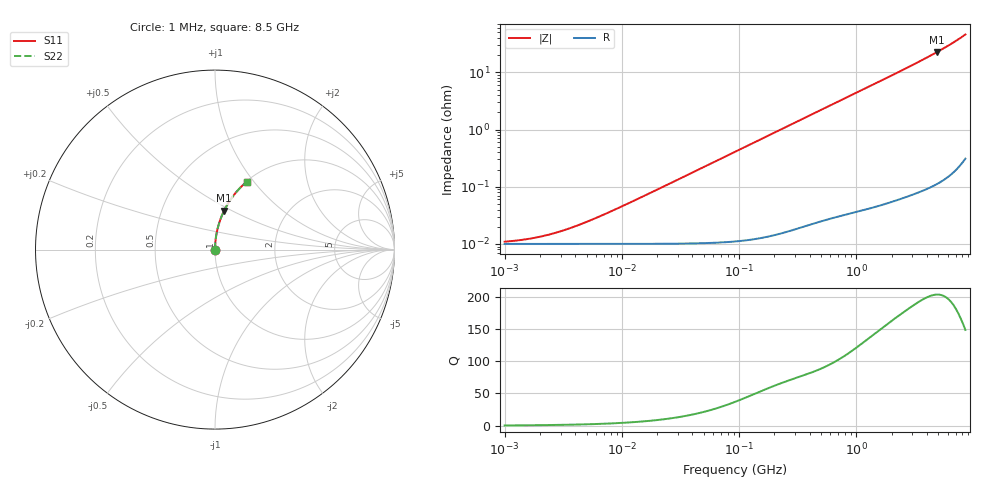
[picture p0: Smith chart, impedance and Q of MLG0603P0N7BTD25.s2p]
! S-Parameter Data Generated by TDK Corporation
! Copyright(C) 2025 TDK Corporation.
! All Rights Reserved.
! TDK P/N: MLG0603P0N7BTD25 (SMD / SMT Inductor (Coil))
! Property: L=0.7nH at 500MHz
! Size(LxWxT): 0.6x0.3x0.3mm
! Model Type: s2p (Touchstone File Format Version 1.0)
! Frequency: DC=Yes Start=1MHz Stop=8500MHz 198points Log-sweep
! Model Generated on Feb. 6, 2025
! Terms and conditions regarding TDK Simulation Models:
! 1)This simulation model is being provided solely for informational
!  purposes. Please refer to the specifications of the products in
!  terms of detailed characteristics of such products.
! 2)In no event shall TDK Corporation of any of its subsidiaries be
!  liable for any loss or damage arising, directly or indirectly,
!  from any information contained in this simulation model, including,
!  but not limited to loss or damages arising from any inaccuracies,
!  omissions or errors in connection with such information.
! 3)Any and all copyrights on this simulation model are owned by
!  TDK Corporation.  Duplication or redistribution of this simulation
!  model without prior written permission from TDK Corporation
!  is prohibited.
! 4)This simulation model is subject to any modification or change
!  without any prior notice.
! 5)Neither TDK Corporation nor any of its subsidiaries shall make any
!  warranty, express or implied, including but not limited to the
!  correctness, implied warranties of merchantability and fitness for
!  a particular purpose with respect to this simulation models.
! 6)The use of this simulation model shall be deemed to have consented
!  to the terms and conditions hereof.
! Port Assignments:
!  1 ---@@@--- 2
! Applicable Conditions:
!  Temperature = 25 degC
!  DC Bias Current = 0 A
!  Small Signal Operation
# Hz S MA R 50
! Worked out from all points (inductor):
!   197 points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, 1 MHz to 8.5 GHz, reference 50 ohm
!   read as one part in series: L = 704 pH near 6.951 MHz
!   highest Q = 203 at 4.885 GHz (marker M1), where L = 742 pH
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1000000  0.0001093 23.9  0.9999 -0.0  0.9999 -0.0  0.0001093 23.9
1515069  0.0001204 33.8  0.9999 -0.0  0.9999 -0.0  0.0001204 33.8
1822320  0.0001285 38.9  0.9999 -0.0  0.9999 -0.0  0.0001285 38.9
2191881  0.0001393 44.1  0.9999 -0.0  0.9999 -0.0  0.0001393 44.1
2636387  0.0001536 49.4  0.9999 -0.0  0.9999 -0.0  0.0001536 49.4
3171038  0.0001723 54.5  0.9999 -0.0  0.9999 -0.0  0.0001723 54.5
4587603  0.0002263 63.8  0.9999 -0.0  0.9999 -0.0  0.0002263 63.8
6051655  0.0002858 69.5  0.9999 -0.0  0.9999 -0.0  0.0002858 69.5
8360083  0.0003832 74.8  0.9999 -0.0  0.9999 -0.0  0.0003832 74.8
2.10461e7  0.0009366 83.8  0.9999 -0.1  0.9999 -0.1  0.0009366 83.8
9.219544e7  0.004079 88.2  0.9999 -0.2  0.9999 -0.2  0.004079 88.2
4.229561e8  0.01861 88.2  0.9996 -1.1  0.9996 -1.1  0.01861 88.2
1.016736e9  0.04459 87.0  0.9986 -2.6  0.9986 -2.6  0.04459 87.0
1.940355e9  0.0853 84.8  0.9958 -4.9  0.9958 -4.9  0.0853 84.8
2.559585e9  0.113 83.2  0.993 -6.5  0.993 -6.5  0.113 83.2
3.224109e9  0.1432 81.5  0.9889 -8.2  0.9889 -8.2  0.1432 81.5
4.061159e9  0.1821 79.2  0.9824 -10.5  0.9824 -10.5  0.1821 79.2
4.884749e9  0.2218 76.9  0.974 -12.8  0.974 -12.8  0.2218 76.9
5.87536e9  0.2715 74.0  0.9611 -15.8  0.9611 -15.8  0.2715 74.0
6.748056e9  0.3176 71.2  0.9465 -18.5  0.9465 -18.5  0.3176 71.2
7.750377e9  0.3735 67.7  0.9254 -21.9  0.9254 -21.9  0.3735 67.7
8.5e9  0.4174 64.9  0.9059 -24.7  0.9059 -24.7  0.4174 64.9
